(* Logix 5000 AddOnInstructionDefinition export FB_SCTMi_IOL; software revision 30.00 *)

TYPE stSCTMi_Ejector :
STRUCT
   siErrorByte : SINT;
   siWarningByte : SINT;
   siLeakageOfLastCycle : SINT;
   iSystemVacuum : INT;
   iEvacuationTimeT1 : INT;
   iLastFreeFlowVacuum : INT;
   iAirConsumptionOfLastCyc : INT;
   bAirSavingFunktion_H1 : BOOL;
   bPartPresent_H2 : BOOL;
END_STRUCT
END_TYPE

ADD_ON_INSTRUCTION FB_SCTMi_IOL   (* revision 1.0, vendor J. Schmalz GmbH *)
VAR_INPUT
   iInputPressure : INT; {access None, visible}
   bVacOnEjector1 : BOOL; {access None, visible}
   bBlowOffEjector1 : BOOL; {access None, visible}
   bVacOnEjector2 : BOOL; {access None, visible}
   bBlowOffEjector2 : BOOL; {access None, visible}
   bVacOnEjector3 : BOOL; {access None, visible}
   bBlowOffEjector3 : BOOL; {access None, visible}
   bVacOnEjector4 : BOOL; {access None, visible}
   bBlowOffEjector4 : BOOL; {access None, visible}
   bVacOnEjector5 : BOOL; {access None, visible}
   bBlowOffEjector5 : BOOL; {access None, visible}
   bVacOnEjector6 : BOOL; {access None, visible}
   bBlowOffEjector6 : BOOL; {access None, visible}
   bVacOnEjector7 : BOOL; {access None, visible}
   bBlowOffEjector7 : BOOL; {access None, visible}
   bVacOnEjector8 : BOOL; {access None, visible}
   bBlowOffEjector8 : BOOL; {access None, visible}
   bVacOnEjector9 : BOOL; {access None, visible}
   bBlowOffEjector9 : BOOL; {access None, visible}
   bVacOnEjector10 : BOOL; {access None, visible}
   bBlowOffEjector10 : BOOL; {access None, visible}
   bVacOnEjector11 : BOOL; {access None, visible}
   bBlowOffEjector11 : BOOL; {access None, visible}
   bVacOnEjector12 : BOOL; {access None, visible}
   bBlowOffEjector12 : BOOL; {access None, visible}
   bVacOnEjector13 : BOOL; {access None, visible}
   bBlowOffEjector13 : BOOL; {access None, visible}
   bVacOnEjector14 : BOOL; {access None, visible}
   bBlowOffEjector14 : BOOL; {access None, visible}
   bVacOnEjector15 : BOOL; {access None, visible}
   bBlowOffEjector15 : BOOL; {access None, visible}
   bVacOnEjector16 : BOOL; {access None, visible}
   bBlowOffEjector16 : BOOL; {access None, visible}
   iNumberOfEjectors : INT; {visible}
   iValveTypes : INT; {visible}
   siPDIData0 : SINT; {visible}
   siPDIData1 : SINT; {visible}
   siPDIData2 : SINT; {visible}
   siPDIData3 : SINT; {visible}
   siPDIData4 : SINT; {visible}
   siPDIData5 : SINT; {visible}
   siPDIData6 : SINT; {visible}
   siPDIData7 : SINT; {visible}
END_VAR
VAR_OUTPUT
   bDeviceStateGreen : BOOL; {visible}
   bDeviceStateYellow : BOOL; {visible}
   bDeviceStateOrange : BOOL; {visible}
   bDeviceStateRed : BOOL; {visible}
   siErrorByteCU : SINT; {visible}
   siWarningByteCU : SINT; {visible}
   iPrimSupplyVoltageCU : INT; {visible}
   iAuxSupplyVoltageCU : INT; {visible}
   iTotalAirConsCU : INT; {visible}
   siPDOData0 : SINT; {visible}
   siPDOData1 : SINT; {visible}
   siPDOData2 : SINT; {visible}
   siPDOData3 : SINT; {visible}
   siPDOData4 : SINT; {visible}
   siPDOData5 : SINT; {visible}
END_VAR
VAR_IN_OUT
   stDataEjector1To16 : stSCTMi_Ejector[16]; {required}
END_VAR
VAR
   iStep : INT; {access None}
   iBuffer0 : INT; {access None}
   iBuffer1 : INT; {access None}
END_VAR

ROUTINE Logic   (* structured text *)
   (*////////////////////////////////////////////////////////////////////////////////////////////////////////////////////////////////////////////////////////////////////
   // -------------------------------------------------------------------------------------------------------------------------------------------------------------------
   // Copyright (C) - J. Schmalz GmbH 2018 -  All rights reserved
   // Subject to change without notice
   // -------------------------------------------------------------------------------------------------------------------------------------------------------------------
   // This function block controls a Schmalz SCTMi-IOL via the process data. With this function block all possible
   // Combinations of ejectors can be controlled.
   // For further information on how the module must be parameterized can be found in the function block documentation.
   // -------------------------------------------------------------------------------------------------------------------------------------------------------------------
   // Version:			1.0
   // Issue Date:		2018-07-20
   // -------------------------------------------------------------------------------------------------------------------------------------------------------------------
   /////////////////////////////////////////////////////////////////////////////////////////////////////////////////////////////////////////////////////////////////////*)
   
   IF EnableIn THEN
   
   (*Sequence: Read epc values*)
   	CASE iStep OF
   
   (* Control Unit *)
   	0:
   		siPDOData0.0:=0;
   		siPDOData0.1:=0;
   		siPDOData0.2:=0;
   		siPDOData0.3:=0;
   		siPDOData0.4:=0;
   
   (* EPC-Value 0 *)
   		siPDOData0.6 := 0;
   		siPDOData0.7 := 0;
   		IF NOT siPDIData0.5  THEN
   			siErrorByteCU := siPDIData1;
   			iBuffer0 := siPDIData3;
   			iBuffer1 := siPDIData2 * 256;
   			iPrimSupplyVoltageCU := iBuffer1 OR iBuffer0;
   			iBuffer0 := 0;
   			iBuffer1 := 0;
   			iStep := iStep + 1;
   		END_IF;
   
   (* EPC-Value 1 *)
   	1:
   		siPDOData0.6 := 1;
   		siPDOData0.7 := 0;
   		IF siPDIData0.5  THEN
   			siWarningByteCU := siPDIData1;
   			iBuffer0 := siPDIData3;
   			iBuffer1 := siPDIData2 * 256;
   			iAuxSupplyVoltageCU := iBuffer1 OR iBuffer0;
   			iBuffer0 := 0;
   			iBuffer1 := 0;
   			iStep := iStep + 1;
   		END_IF;
   
   (* intermediate step *)
   	2:
   		siPDOData0.6 := 0;
   		siPDOData0.7 := 0;
   		IF NOT siPDIData0.5  THEN
   			iStep := iStep + 1;
   		END_IF;
   
   (* EPC-Value 2 *)
   	3:
   		siPDOData0.6 := 0;
   		siPDOData0.7 := 1;
   		IF siPDIData0.5  THEN
   			iStep := iStep + 1;
   		END_IF;
   
   (* intermediate step *)
   	4:
   		siPDOData0.6 := 0;
   		siPDOData0.7 := 0;
   		IF NOT siPDIData0.5  THEN
   			iStep := iStep + 1;
   		END_IF;
   
   (* EPC-Value 3 *)
   	5:
   		siPDOData0.6 := 1;
   		siPDOData0.7 := 1;
   		IF siPDIData0.5  THEN
   			iBuffer0 := siPDIData3;
   			iBuffer1 := siPDIData2 * 256;
   			iTotalAirConsCU := iBuffer1 OR iBuffer0;
   			iBuffer0 := 0;
   			iBuffer1 := 0;
   			iStep := iStep + 1;
   		END_IF;
   
   	6:
   			IF iNumberOfEjectors >= 1 THEN
   				iStep := iStep + 1;
   			ELSE
   				iStep:= 0;
   			END_IF;
   
   (* Ejector 1 *)
   	7:
   		siPDOData0.0:=1;
   		siPDOData0.1:=0;
   		siPDOData0.2:=0;
   		siPDOData0.3:=0;
   		siPDOData0.4:=0;
   
   (* EPC-Value 0 *)
   		siPDOData0.6 := 0;
   		siPDOData0.7 := 0;
   		IF NOT siPDIData0.5  THEN
   			stDataEjector1To16[0].siErrorByte := siPDIData1;
   			iBuffer0 := siPDIData3;
   			iBuffer1 := siPDIData2 * 256;
   			stDataEjector1To16[0].iSystemVacuum:= iBuffer1 OR iBuffer0;
   			iBuffer0 := 0;
   			iBuffer1 := 0;
   			iStep := iStep + 1;
   		END_IF;
   
   (* EPC-Value 1 *)
   	8:
   		siPDOData0.6 := 1;
   		siPDOData0.7 := 0;
   		IF siPDIData0.5  THEN
   			stDataEjector1To16[0].siWarningByte := siPDIData1;
   			iBuffer0 := siPDIData3;
   			iBuffer1 := siPDIData2 * 256;
   			stDataEjector1To16[0].iEvacuationTimeT1 := iBuffer1 OR iBuffer0;
   			iBuffer0 := 0;
   			iBuffer1 := 0;
   			iStep := iStep + 1;
   		END_IF;
   
   (* intermediate step *)
   	9:
   		siPDOData0.6 := 0;
   		siPDOData0.7 := 0;
   		IF NOT siPDIData0.5  THEN
   			iStep := iStep + 1;
   		END_IF;
   
   (* EPC-Value 2 *)
   	10:
   		siPDOData0.6 := 0;
   		siPDOData0.7 := 1;
   		IF siPDIData0.5  THEN
   			iBuffer0 := siPDIData3;
   			iBuffer1 := siPDIData2 * 256;
   			stDataEjector1To16[0].iLastFreeFlowVacuum := iBuffer1 OR iBuffer0;
   			iBuffer0 := 0;
   			iBuffer1 := 0;
   			iStep := iStep + 1;
   		END_IF;
   
   (* intermediate step *)
   	11:
   		siPDOData0.6 := 0;
   		siPDOData0.7 := 0;
   		IF NOT siPDIData0.5  THEN
   			iStep := iStep + 1;
   		END_IF;
   
    (* EPC-Value 3 *)
   	12:
   		siPDOData0.6 := 1;
   		siPDOData0.7 := 1;
   		IF siPDIData0.5  THEN
   			stDataEjector1To16[0].siLeakageOfLastCycle := siPDIData1;
   			iBuffer0 := siPDIData3;
   			iBuffer1 := siPDIData2 * 256;
   			stDataEjector1To16[0].iAirConsumptionOfLastCyc := iBuffer1 OR iBuffer0;
   			iBuffer0 := 0;
   			iBuffer1 := 0;
   			iStep := iStep + 1;
   		END_IF;
   
   	13:
   		IF iNumberOfEjectors >= 2 THEN
   			iStep := iStep + 1;
   		ELSE
   			iStep:= 0;
   		END_IF;
   
   (* Ejector 2 *)
   	14:
   		siPDOData0.0:=0;
   		siPDOData0.1:=1;
   		siPDOData0.2:=0;
   		siPDOData0.3:=0;
   		siPDOData0.4:=0;
   
   (* EPC-Value 0 *)
   		siPDOData0.6 := 0;
   		siPDOData0.7 := 0;
   		IF NOT siPDIData0.5  THEN
   			stDataEjector1To16[1].siErrorByte := siPDIData1;
   			iBuffer0 := siPDIData3;
   			iBuffer1 := siPDIData2 * 256;
   			stDataEjector1To16[1].iSystemVacuum:= iBuffer1 OR iBuffer0;
   			iBuffer0 := 0;
   			iBuffer1 := 0;
   			iStep := iStep + 1;
   		END_IF;
   
   (* EPC-Value 1 *)
   	15:
   		siPDOData0.6 := 1;
   		siPDOData0.7 := 0;
   		IF siPDIData0.5  THEN
   			stDataEjector1To16[1].siWarningByte := siPDIData1;
   			iBuffer0 := siPDIData3;
   			iBuffer1 := siPDIData2 * 256;
   			stDataEjector1To16[1].iEvacuationTimeT1 := iBuffer1 OR iBuffer0;
   			iBuffer0 := 0;
   			iBuffer1 := 0;
   			iStep := iStep + 1;
   		END_IF;
   
   (* intermediate step *)
   	16:
   		siPDOData0.6 := 0;
   		siPDOData0.7 := 0;
   		IF NOT siPDIData0.5  THEN
   			iStep := iStep + 1;
   		END_IF;
   
   (* EPC-Value 2 *)
   	17:
   		siPDOData0.6 := 0;
   		siPDOData0.7 := 1;
   		IF siPDIData0.5  THEN
   			iBuffer0 := siPDIData3;
   			iBuffer1 := siPDIData2 * 256;
   			stDataEjector1To16[1].iLastFreeFlowVacuum := iBuffer1 OR iBuffer0;
   			iBuffer0 := 0;
   			iBuffer1 := 0;
   			iStep := iStep + 1;
   		END_IF;
   
   (* intermediate step *)
   	18:
   		siPDOData0.6 := 0;
   		siPDOData0.7 := 0;
   		IF NOT siPDIData0.5  THEN
   			iStep := iStep + 1;
   		END_IF;
   
   (* EPC-Value 3 *)
   	19:	(* EPC-Value 3 *)
   		siPDOData0.6 := 1;
   		siPDOData0.7 := 1;
   		IF siPDIData0.5  THEN
   			stDataEjector1To16[1].siLeakageOfLastCycle := siPDIData1;
   			iBuffer0 := siPDIData3;
   			iBuffer1 := siPDIData2 * 256;
   			stDataEjector1To16[1].iAirConsumptionOfLastCyc := iBuffer1 OR iBuffer0;
   			iBuffer0 := 0;
   			iBuffer1 := 0;
   			iStep := iStep + 1;
   		END_IF;
   
   	20:
   		IF iNumberOfEjectors >= 3 THEN
   			iStep := iStep + 1;
   		ELSE
   			iStep:= 0;
   		END_IF;
   
   (* Ejector 3 *)
   	21:
   		siPDOData0.0:=1;
   		siPDOData0.1:=1;
   		siPDOData0.2:=0;
   		siPDOData0.3:=0;
   		siPDOData0.4:=0;
   
   (* EPC-Value 0 *)
   		siPDOData0.6 := 0;
   		siPDOData0.7 := 0;
   		IF NOT siPDIData0.5  THEN
   			stDataEjector1To16[2].siErrorByte := siPDIData1;
   			iBuffer0 := siPDIData3;
   			iBuffer1 := siPDIData2 * 256;
   			stDataEjector1To16[2].iSystemVacuum:= iBuffer1 OR iBuffer0;
   			iBuffer0 := 0;
   			iBuffer1 := 0;
   			iStep := iStep + 1;
   		END_IF;
   
   (* EPC-Value 1 *)
   	22:
   		siPDOData0.6 := 1;
   		siPDOData0.7 := 0;
   		IF siPDIData0.5  THEN
   			stDataEjector1To16[2].siWarningByte := siPDIData1;
   			iBuffer0 := siPDIData3;
   			iBuffer1 := siPDIData2 * 256;
   			stDataEjector1To16[2].iEvacuationTimeT1 := iBuffer1 OR iBuffer0;
   			iBuffer0 := 0;
   			iBuffer1 := 0;
   			iStep := iStep + 1;
   		END_IF;
   
   (* intermediate step *)
   	23:
   		siPDOData0.6 := 0;
   		siPDOData0.7 := 0;
   		IF NOT siPDIData0.5  THEN
   			iStep := iStep + 1;
   		END_IF;
   
   (* EPC-Value 2 *)
   	24:
   		siPDOData0.6 := 0;
   		siPDOData0.7 := 1;
   		IF siPDIData0.5  THEN
   			iBuffer0 := siPDIData3;
   			iBuffer1 := siPDIData2 * 256;
   			stDataEjector1To16[2].iLastFreeFlowVacuum := iBuffer1 OR iBuffer0;
   			iBuffer0 := 0;
   			iBuffer1 := 0;
   			iStep := iStep + 1;
   		END_IF;
   
   (* intermediate step *)
   	25:
   		siPDOData0.6 := 0;
   		siPDOData0.7 := 0;
   		IF NOT siPDIData0.5  THEN
   			iStep := iStep + 1;
   		END_IF;
   
   (* EPC-Value 3 *)
   	26:
   		siPDOData0.6 := 1;
   		siPDOData0.7 := 1;
   		IF siPDIData0.5  THEN
   			stDataEjector1To16[2].siLeakageOfLastCycle := siPDIData1;
   			iBuffer0 := siPDIData3;
   			iBuffer1 := siPDIData2 * 256;
   			stDataEjector1To16[2].iAirConsumptionOfLastCyc := iBuffer1 OR iBuffer0;
   			iBuffer0 := 0;
   			iBuffer1 := 0;
   			iStep := iStep + 1;
   		END_IF;
   
   	27:
   		IF iNumberOfEjectors >= 4 THEN
   			iStep := iStep + 1;
   		ELSE
   			iStep:= 0;
   		END_IF;
   
   (* Ejector 4 *)
   	28:
   		siPDOData0.0:=0;
   		siPDOData0.1:=0;
   		siPDOData0.2:=1;
   		siPDOData0.3:=0;
   		siPDOData0.4:=0;
   
   (* EPC-Value 0 *)
   		siPDOData0.6 := 0;
   		siPDOData0.7 := 0;
   		IF NOT siPDIData0.5  THEN
   			stDataEjector1To16[3].siErrorByte := siPDIData1;
   			iBuffer0 := siPDIData3;
   			iBuffer1 := siPDIData2 * 256;
   			stDataEjector1To16[3].iSystemVacuum := iBuffer1 OR iBuffer0;
   			iBuffer0 := 0;
   			iBuffer1 := 0;
   			iStep := iStep + 1;
   		END_IF;
   
   (* EPC-Value 1 *)
   	29:
   		siPDOData0.6 := 1;
   		siPDOData0.7 := 0;
   		IF siPDIData0.5  THEN
   			stDataEjector1To16[3].siWarningByte := siPDIData1;
   			iBuffer0 := siPDIData3;
   			iBuffer1 := siPDIData2 * 256;
   			stDataEjector1To16[3].iEvacuationTimeT1 := iBuffer1 OR iBuffer0;
   			iBuffer0 := 0;
   			iBuffer1 := 0;
   			iStep := iStep + 1;
   		END_IF;
   
   (* intermediate step *)
   	30:
   		siPDOData0.6 := 0;
   		siPDOData0.7 := 0;
   		IF NOT siPDIData0.5  THEN
   			iStep := iStep + 1;
   		END_IF;
   
   (* EPC-Value 2 *)
   	31:
   		siPDOData0.6 := 0;
   		siPDOData0.7 := 1;
   		IF siPDIData0.5  THEN
   			iBuffer0 := siPDIData3;
   			iBuffer1 := siPDIData2 * 256;
   			stDataEjector1To16[3].iLastFreeFlowVacuum := iBuffer1 OR iBuffer0;
   			iBuffer0 := 0;
   			iBuffer1 := 0;
   			iStep := iStep + 1;
   		END_IF;
   
   (* intermediate step *)
   	32:
   		siPDOData0.6 := 0;
   		siPDOData0.7 := 0;
   		IF NOT siPDIData0.5  THEN
   			iStep := iStep + 1;
   		END_IF;
   
   (* EPC-Value 3 *)
   	33:
   		siPDOData0.6 := 1;
   		siPDOData0.7 := 1;
   		IF siPDIData0.5  THEN
   			stDataEjector1To16[3].siLeakageOfLastCycle := siPDIData1;
   			iBuffer0 := siPDIData3;
   			iBuffer1 := siPDIData2 * 256;
   			stDataEjector1To16[3].iAirConsumptionOfLastCyc := iBuffer1 OR iBuffer0;
   			iBuffer0 := 0;
   			iBuffer1 := 0;
   			iStep := iStep + 1;
   		END_IF;
   
   	34:
   		IF iNumberOfEjectors >= 5 THEN
   			iStep := iStep + 1;
   		ELSE
   			iStep:= 0;
   		END_IF;
   
   
   (* Ejector 5 *)
   	35:
   		siPDOData0.0:=1;
   		siPDOData0.1:=0;
   		siPDOData0.2:=1;
   		siPDOData0.3:=0;
   		siPDOData0.4:=0;
   
   (* EPC-Value 0 *)
   		siPDOData0.6 := 0;
   		siPDOData0.7 := 0;
   		IF NOT siPDIData0.5  THEN
   			stDataEjector1To16[4].siErrorByte := siPDIData1;
   			iBuffer0 := siPDIData3;
   			iBuffer1 := siPDIData2 * 256;
   			stDataEjector1To16[4].iSystemVacuum:= iBuffer1 OR iBuffer0;
   			iBuffer0 := 0;
   			iBuffer1 := 0;
   			iStep := iStep + 1;
   		END_IF;
   
   (* EPC-Value 1 *)
   	36:
   		siPDOData0.6 := 1;
   		siPDOData0.7 := 0;
   		IF siPDIData0.5  THEN
   			stDataEjector1To16[4].siWarningByte := siPDIData1;
   			iBuffer0 := siPDIData3;
   			iBuffer1 := siPDIData2 * 256;
   			stDataEjector1To16[4].iEvacuationTimeT1 := iBuffer1 OR iBuffer0;
   			iBuffer0 := 0;
   			iBuffer1 := 0;
   			iStep := iStep + 1;
   		END_IF;
   
   (* intermediate step *)
   	37:
   		siPDOData0.6 := 0;
   		siPDOData0.7 := 0;
   		IF NOT siPDIData0.5  THEN
   			iStep := iStep + 1;
   		END_IF;
   
   (* EPC-Value 2 *)
   	38:
   		siPDOData0.6 := 0;
   		siPDOData0.7 := 1;
   		IF siPDIData0.5  THEN
   			iBuffer0 := siPDIData3;
   			iBuffer1 := siPDIData2 * 256;
   			stDataEjector1To16[4].iLastFreeFlowVacuum := iBuffer1 OR iBuffer0;
   			iBuffer0 := 0;
   			iBuffer1 := 0;
   			iStep := iStep + 1;
   		END_IF;
   
   (* intermediate step *)
   	39:
   		siPDOData0.6 := 0;
   		siPDOData0.7 := 0;
   		IF NOT siPDIData0.5  THEN
   			iStep := iStep + 1;
   		END_IF;
   
   (* EPC-Value 3 *)
   	40:
   		siPDOData0.6 := 1;
   		siPDOData0.7 := 1;
   		IF siPDIData0.5  THEN
   			stDataEjector1To16[4].siLeakageOfLastCycle := siPDIData1;
   			iBuffer0 := siPDIData3;
   			iBuffer1 := siPDIData2 * 256;
   			stDataEjector1To16[4].iAirConsumptionOfLastCyc := iBuffer1 OR iBuffer0;
   			iBuffer0 := 0;
   			iBuffer1 := 0;
   			iStep := iStep + 1;
   		END_IF;
   
   	41:
   		IF iNumberOfEjectors >= 6 THEN
   			iStep := iStep + 1;
   		ELSE
   			iStep:= 0;
   		END_IF;
   
   (* Ejector 6 *)
   	42:
   		siPDOData0.0:=0;
   		siPDOData0.1:=1;
   		siPDOData0.2:=1;
   		siPDOData0.3:=0;
   		siPDOData0.4:=0;
   
   (* EPC-Value 0 *)
   		siPDOData0.6 := 0;
   		siPDOData0.7 := 0;
   		IF NOT siPDIData0.5  THEN
   			stDataEjector1To16[5].siErrorByte := siPDIData1;
   			iBuffer0 := siPDIData3;
   			iBuffer1 := siPDIData2 * 256;
   			stDataEjector1To16[5].iSystemVacuum:= iBuffer1 OR iBuffer0;
   			iBuffer0 := 0;
   			iBuffer1 := 0;
   			iStep := iStep + 1;
   		END_IF;
   
   (* EPC-Value 1 *)
   	43:
   		siPDOData0.6 := 1;
   		siPDOData0.7 := 0;
   		IF siPDIData0.5  THEN
   			stDataEjector1To16[5].siWarningByte := siPDIData1;
   			iBuffer0 := siPDIData3;
   			iBuffer1 := siPDIData2 * 256;
   			stDataEjector1To16[5].iEvacuationTimeT1 := iBuffer1 OR iBuffer0;
   			iBuffer0 := 0;
   			iBuffer1 := 0;
   			iStep := iStep + 1;
   		END_IF;
   
   (* intermediate step *)
   	44:
   		siPDOData0.6 := 0;
   		siPDOData0.7 := 0;
   
   		IF NOT siPDIData0.5  THEN
   			iStep := iStep + 1;
   		END_IF;
   
   (* EPC-Value 2 *)
   	45:
   		siPDOData0.6 := 0;
   		siPDOData0.7 := 1;
   		IF siPDIData0.5  THEN
   			iBuffer0 := siPDIData3;
   			iBuffer1 := siPDIData2 * 256;
   			stDataEjector1To16[5].iLastFreeFlowVacuum := iBuffer1 OR iBuffer0;
   			iBuffer0 := 0;
   			iBuffer1 := 0;
   			iStep := iStep + 1;
   		END_IF;
   
   (* intermediate step *)
   	46:
   		siPDOData0.6 := 0;
   		siPDOData0.7 := 0;
   		IF NOT siPDIData0.5  THEN
   			iStep := iStep + 1;
   		END_IF;
   
   (* EPC-Value 3 *)
   	47:
   		siPDOData0.6 := 1;
   		siPDOData0.7 := 1;
   		IF siPDIData0.5  THEN
   			stDataEjector1To16[5].siLeakageOfLastCycle := siPDIData1;
   			iBuffer0 := siPDIData3;
   			iBuffer1 := siPDIData2 * 256;
   			stDataEjector1To16[5].iAirConsumptionOfLastCyc := iBuffer1 OR iBuffer0;
   			iBuffer0 := 0;
   			iBuffer1 := 0;
   			iStep := iStep + 1;
   		END_IF;
   
   	48:
   		IF iNumberOfEjectors >= 7 THEN
   			iStep := iStep + 1;
   		ELSE
   			iStep:= 0;
   		END_IF;
   
   (* Ejector 7 *)
   	49:
   		siPDOData0.0:=1;
   		siPDOData0.1:=1;
   		siPDOData0.2:=1;
   		siPDOData0.3:=0;
   		siPDOData0.4:=0;
   
   (* EPC-Value 0 *)
   		siPDOData0.6 := 0;
   		siPDOData0.7 := 0;
   		IF NOT siPDIData0.5  THEN
   			stDataEjector1To16[6].siErrorByte := siPDIData1;
   			iBuffer0 := siPDIData3;
   			iBuffer1 := siPDIData2 * 256;
   			stDataEjector1To16[6].iSystemVacuum:= iBuffer1 OR iBuffer0;
   			iBuffer0 := 0;
   			iBuffer1 := 0;
   			iStep := iStep + 1;
   		END_IF;
   
   (* EPC-Value 1 *)
   	50:
   		siPDOData0.6 := 1;
   		siPDOData0.7 := 0;
   		IF siPDIData0.5  THEN
   			stDataEjector1To16[6].siWarningByte := siPDIData1;
   			iBuffer0 := siPDIData3;
   			iBuffer1 := siPDIData2 * 256;
   			stDataEjector1To16[6].iEvacuationTimeT1 := iBuffer1 OR iBuffer0;
   			iBuffer0 := 0;
   			iBuffer1 := 0;
   			iStep := iStep + 1;
   		END_IF;
   
   (* intermediate step *)
   	51:
   		siPDOData0.6 := 0;
   		siPDOData0.7 := 0;
   		IF NOT siPDIData0.5  THEN
   			iStep := iStep + 1;
   		END_IF;
   
   (* EPC-Value 2 *)
   	52:
   		siPDOData0.6 := 0;
   		siPDOData0.7 := 1;
   		IF siPDIData0.5  THEN
   			iBuffer0 := siPDIData3;
   			iBuffer1 := siPDIData2 * 256;
   			stDataEjector1To16[6].iLastFreeFlowVacuum := iBuffer1 OR iBuffer0;
   			iBuffer0 := 0;
   			iBuffer1 := 0;
   			iStep := iStep + 1;
   		END_IF;
   
   (* intermediate step *)
   	53:
   		siPDOData0.6 := 0;
   		siPDOData0.7 := 0;
   		IF NOT siPDIData0.5  THEN
   			iStep := iStep + 1;
   		END_IF;
   
   (* EPC-Value 3 *)
   	54:
   		siPDOData0.6 := 1;
   		siPDOData0.7 := 1;
   		IF siPDIData0.5  THEN
   			stDataEjector1To16[6].siLeakageOfLastCycle := siPDIData1;
   			iBuffer0 := siPDIData3;
   			iBuffer1 := siPDIData2 * 256;
   			stDataEjector1To16[6].iAirConsumptionOfLastCyc := iBuffer1 OR iBuffer0;
   			iBuffer0 := 0;
   			iBuffer1 := 0;
   			iStep := iStep + 1;
   		END_IF;
   
   	55:
   		IF iNumberOfEjectors >= 8 THEN
   			iStep := iStep + 1;
   		ELSE
   			iStep:= 0;
   		END_IF;
   
   (* Ejector 8 *)
   	56:
   		siPDOData0.0:=0;
   		siPDOData0.1:=0;
   		siPDOData0.2:=0;
   		siPDOData0.3:=1;
   		siPDOData0.4:=0;
   
   (* EPC-Value 0 *)
   		siPDOData0.6 := 0;
   		siPDOData0.7 := 0;
   		IF NOT siPDIData0.5  THEN
   			stDataEjector1To16[7].siErrorByte := siPDIData1;
   			iBuffer0 := siPDIData3;
   			iBuffer1 := siPDIData2 * 256;
   			stDataEjector1To16[7].iSystemVacuum:= iBuffer1 OR iBuffer0;
   			iBuffer0 := 0;
   			iBuffer1 := 0;
   			iStep := iStep + 1;
   		END_IF;
   
   (* EPC-Value 1 *)
   	57:
   		siPDOData0.6 := 1;
   		siPDOData0.7 := 0;
   		IF siPDIData0.5  THEN
   			stDataEjector1To16[7].siWarningByte := siPDIData1;
   			iBuffer0 := siPDIData3;
   			iBuffer1 := siPDIData2 * 256;
   			stDataEjector1To16[7].iEvacuationTimeT1 := iBuffer1 OR iBuffer0;
   			iBuffer0 := 0;
   			iBuffer1 := 0;
   			iStep := iStep + 1;
   		END_IF;
   
   (* intermediate step *)
   	58:
   		siPDOData0.6 := 0;
   		siPDOData0.7 := 0;
   		IF NOT siPDIData0.5  THEN
   			iStep := iStep + 1;
   		END_IF;
   
   (* EPC-Value 2 *)
   	59:
   		siPDOData0.6 := 0;
   		siPDOData0.7 := 1;
   		IF siPDIData0.5  THEN
   			iBuffer0 := siPDIData3;
   			iBuffer1 := siPDIData2 * 256;
   			stDataEjector1To16[7].iLastFreeFlowVacuum := iBuffer1 OR iBuffer0;
   			iBuffer0 := 0;
   			iBuffer1 := 0;
   			iStep := iStep + 1;
   		END_IF;
   
   (* intermediate step *)
   	60:
   		siPDOData0.6 := 0;
   		siPDOData0.7 := 0;
   		IF NOT siPDIData0.5  THEN
   			iStep := iStep + 1;
   		END_IF;
   
   (* EPC-Value 3 *)
   	61:
   		siPDOData0.6 := 1;
   		siPDOData0.7 := 1;
   		IF siPDIData0.5  THEN
   			stDataEjector1To16[7].siLeakageOfLastCycle := siPDIData1;
   			iBuffer0 := siPDIData3;
   			iBuffer1 := siPDIData2 * 256;
   			stDataEjector1To16[7].iAirConsumptionOfLastCyc := iBuffer1 OR iBuffer0;
   			iBuffer0 := 0;
   			iBuffer1 := 0;
   			iStep := iStep + 1;
   		END_IF;
   
   	62:
   		IF iNumberOfEjectors >= 9 THEN
   			iStep := iStep + 1;
   		ELSE
   			iStep:= 0;
   		END_IF;
   
   (* Ejector 9 *)
   	63:
   		siPDOData0.0:=1;
   		siPDOData0.1:=0;
   		siPDOData0.2:=0;
   		siPDOData0.3:=1;
   		siPDOData0.4:=0;
   
   (* EPC-Value 0 *)
   		siPDOData0.6 := 0;
   		siPDOData0.7 := 0;
   		IF NOT siPDIData0.5  THEN
   			stDataEjector1To16[8].siErrorByte := siPDIData1;
   			iBuffer0 := siPDIData3;
   			iBuffer1 := siPDIData2 * 256;
   			stDataEjector1To16[8].iSystemVacuum:= iBuffer1 OR iBuffer0;
   			iBuffer0 := 0;
   			iBuffer1 := 0;
   			iStep := iStep + 1;
   		END_IF;
   
   (* EPC-Value 1 *)
   	64:
   		siPDOData0.6 := 1;
   		siPDOData0.7 := 0;
   		IF siPDIData0.5  THEN
   			stDataEjector1To16[8].siWarningByte := siPDIData1;
   			iBuffer0 := siPDIData3;
   			iBuffer1 := siPDIData2 * 256;
   			stDataEjector1To16[8].iEvacuationTimeT1 := iBuffer1 OR iBuffer0;
   			iBuffer0 := 0;
   			iBuffer1 := 0;
   			iStep := iStep + 1;
   		END_IF;
   
   (* intermediate step *)
   	65:
   		siPDOData0.6 := 0;
   		siPDOData0.7 := 0;
   		IF NOT siPDIData0.5  THEN
   			iStep := iStep + 1;
   		END_IF;
   
   (* EPC-Value 2 *)
   	66:
   		siPDOData0.6 := 0;
   		siPDOData0.7 := 1;
   		IF siPDIData0.5  THEN
   			iBuffer0 := siPDIData3;
   			iBuffer1 := siPDIData2 * 256;
   			stDataEjector1To16[8].iLastFreeFlowVacuum := iBuffer1 OR iBuffer0;
   			iBuffer0 := 0;
   			iBuffer1 := 0;
   			iStep := iStep + 1;
   		END_IF;
   
   (* intermediate step *)
   	67:
   		siPDOData0.6 := 0;
   		siPDOData0.7 := 0;
   		IF NOT siPDIData0.5  THEN
   			iStep := iStep + 1;
   		END_IF;
   
   (* EPC-Value 3 *)
   	68:
   		siPDOData0.6 := 1;
   		siPDOData0.7 := 1;
   		IF siPDIData0.5  THEN
   			stDataEjector1To16[8].siLeakageOfLastCycle := siPDIData1;
   			iBuffer0 := siPDIData3;
   			iBuffer1 := siPDIData2 * 256;
   			stDataEjector1To16[8].iAirConsumptionOfLastCyc := iBuffer1 OR iBuffer0;
   			iBuffer0 := 0;
   			iBuffer1 := 0;
   			iStep := iStep + 1;
   		END_IF;
   
   	69:
   		IF iNumberOfEjectors >= 10 THEN
   			iStep := iStep + 1;
   		ELSE
   			iStep:= 0;
   		END_IF;
   
   (* Ejector 10 *)
   
   	70:
   		siPDOData0.0:=0;
   		siPDOData0.1:=1;
   		siPDOData0.2:=0;
   		siPDOData0.3:=1;
   		siPDOData0.4:=0;
   
   (* EPC-Value 0 *)
   		siPDOData0.6 := 0;
   		siPDOData0.7 := 0;
   		IF NOT siPDIData0.5  THEN
   			stDataEjector1To16[9].siErrorByte := siPDIData1;
   			iBuffer0 := siPDIData3;
   			iBuffer1 := siPDIData2 * 256;
   			stDataEjector1To16[9].iSystemVacuum:= iBuffer1 OR iBuffer0;
   			iBuffer0 := 0;
   			iBuffer1 := 0;
   			iStep := iStep + 1;
   		END_IF;
   
   (* EPC-Value 1 *)
   	71:
   		siPDOData0.6 := 1;
   		siPDOData0.7 := 0;
   		IF siPDIData0.5  THEN
   			stDataEjector1To16[9].siWarningByte := siPDIData1;
   			iBuffer0 := siPDIData3;
   			iBuffer1 := siPDIData2 * 256;
   			stDataEjector1To16[9].iEvacuationTimeT1 := iBuffer1 OR iBuffer0;
   			iBuffer0 := 0;
   			iBuffer1 := 0;
   			iStep := iStep + 1;
   		END_IF;
   
   (* intermediate step *)
   	72:
   		siPDOData0.6 := 0;
   		siPDOData0.7 := 0;
   		IF NOT siPDIData0.5  THEN
   			iStep := iStep + 1;
   		END_IF;
   
   (* EPC-Value 2 *)
   	73:
   		siPDOData0.6 := 0;
   		siPDOData0.7 := 1;
   		IF siPDIData0.5  THEN
   			iBuffer0 := siPDIData3;
   			iBuffer1 := siPDIData2 * 256;
   			stDataEjector1To16[9].iLastFreeFlowVacuum := iBuffer1 OR iBuffer0;
   			iBuffer0 := 0;
   			iBuffer1 := 0;
   			iStep := iStep + 1;
   		END_IF;
   
   (* intermediate step *)
   	74:
   		siPDOData0.6 := 0;
   		siPDOData0.7 := 0;
   		IF NOT siPDIData0.5  THEN
   			iStep := iStep + 1;
   		END_IF;
   
   (* EPC-Value 3 *)
   	75:
   		siPDOData0.6 := 1;
   		siPDOData0.7 := 1;
   		IF siPDIData0.5  THEN
   			stDataEjector1To16[9].siLeakageOfLastCycle := siPDIData1;
   			iBuffer0 := siPDIData3;
   			iBuffer1 := siPDIData2 * 256;
   			stDataEjector1To16[9].iAirConsumptionOfLastCyc := iBuffer1 OR iBuffer0;
   			iBuffer0 := 0;
   			iBuffer1 := 0;
   			iStep := iStep + 1;
   		END_IF;
   
   	76:
   		IF iNumberOfEjectors >= 11 THEN
   			iStep := iStep + 1;
   		ELSE
   			iStep:= 0;
   		END_IF;
   
   (* Ejector 11 *)
   	77:
   		siPDOData0.0:=1;
   		siPDOData0.1:=1;
   		siPDOData0.2:=0;
   		siPDOData0.3:=1;
   		siPDOData0.4:=0;
   
   (* EPC-Value 0 *)
   		siPDOData0.6 := 0;
   		siPDOData0.7 := 0;
   		IF NOT siPDIData0.5  THEN
   			stDataEjector1To16[10].siErrorByte := siPDIData1;
   			iBuffer0 := siPDIData3;
   			iBuffer1 := siPDIData2 * 256;
   			stDataEjector1To16[10].iSystemVacuum:= iBuffer1 OR iBuffer0;
   			iBuffer0 := 0;
   			iBuffer1 := 0;
   			iStep := iStep + 1;
   		END_IF;
   
   (* EPC-Value 1 *)
   	78:
   		siPDOData0.6 := 1;
   		siPDOData0.7 := 0;
   		IF siPDIData0.5  THEN
   			stDataEjector1To16[10].siWarningByte := siPDIData1;
   			iBuffer0 := siPDIData3;
   			iBuffer1 := siPDIData2 * 256;
   			stDataEjector1To16[10].iEvacuationTimeT1 := iBuffer1 OR iBuffer0;
   			iBuffer0 := 0;
   			iBuffer1 := 0;
   			iStep := iStep + 1;
   		END_IF;
   
   (* intermediate step *)
   	79:
   		siPDOData0.6 := 0;
   		siPDOData0.7 := 0;
   		IF NOT siPDIData0.5  THEN
   			iStep := iStep + 1;
   		END_IF;
   
   (* EPC-Value 2 *)
   	80:
   		siPDOData0.6 := 0;
   		siPDOData0.7 := 1;
   		IF siPDIData0.5  THEN
   			iBuffer0 := siPDIData3;
   			iBuffer1 := siPDIData2 * 256;
   			stDataEjector1To16[10].iLastFreeFlowVacuum := iBuffer1 OR iBuffer0;
   			iBuffer0 := 0;
   			iBuffer1 := 0;
   			iStep := iStep + 1;
   		END_IF;
   
   (* intermediate step *)
   	81:
   		siPDOData0.6 := 0;
   		siPDOData0.7 := 0;
   		IF NOT siPDIData0.5  THEN
   			iStep := iStep + 1;
   		END_IF;
   
   (* EPC-Value 3 *)
   	82:
   		siPDOData0.6 := 1;
   		siPDOData0.7 := 1;
   		IF siPDIData0.5  THEN
   			stDataEjector1To16[10].siLeakageOfLastCycle := siPDIData1;
   			iBuffer0 := siPDIData3;
   			iBuffer1 := siPDIData2 * 256;
   			stDataEjector1To16[10].iAirConsumptionOfLastCyc := iBuffer1 OR iBuffer0;
   			iBuffer0 := 0;
   			iBuffer1 := 0;
   			iStep := iStep + 1;
   		END_IF;
   
   	83:
   		IF iNumberOfEjectors >= 12 THEN
   			iStep := iStep + 1;
   		ELSE
   			iStep:= 0;
   		END_IF;
   
   (* Ejector 12 *)
   	84:
   		siPDOData0.0:=0;
   		siPDOData0.1:=0;
   		siPDOData0.2:=1;
   		siPDOData0.3:=1;
   		siPDOData0.4:=0;
   
   (* EPC-Value 0 *)
   		siPDOData0.6 := 0;
   		siPDOData0.7 := 0;
   		IF NOT siPDIData0.5  THEN
   			stDataEjector1To16[11].siErrorByte := siPDIData1;
   			iBuffer0 := siPDIData3;
   			iBuffer1 := siPDIData2 * 256;
   			stDataEjector1To16[11].iSystemVacuum:= iBuffer1 OR iBuffer0;
   			iBuffer0 := 0;
   			iBuffer1 := 0;
   			iStep := iStep + 1;
   		END_IF;
   
   (* EPC-Value 1 *)
   	85:
   		siPDOData0.6 := 1;
   		siPDOData0.7 := 0;
   		IF siPDIData0.5  THEN
   			stDataEjector1To16[11].siWarningByte := siPDIData1;
   			iBuffer0 := siPDIData3;
   			iBuffer1 := siPDIData2 * 256;
   			stDataEjector1To16[11].iEvacuationTimeT1 := iBuffer1 OR iBuffer0;
   			iBuffer0 := 0;
   			iBuffer1 := 0;
   			iStep := iStep + 1;
   		END_IF;
   
   (* intermediate step *)
   	86:
   		siPDOData0.6 := 0;
   		siPDOData0.7 := 0;
   		IF NOT siPDIData0.5  THEN
   			iStep := iStep + 1;
   		END_IF;
   
   (* EPC-Value 2 *)
   	87:
   		siPDOData0.6 := 0;
   		siPDOData0.7 := 1;
   		IF siPDIData0.5  THEN
   			iBuffer0 := siPDIData3;
   			iBuffer1 := siPDIData2 * 256;
   			stDataEjector1To16[11].iLastFreeFlowVacuum := iBuffer1 OR iBuffer0;
   			iBuffer0 := 0;
   			iBuffer1 := 0;
   			iStep := iStep + 1;
   		END_IF;
   
   (* intermediate step *)
   	88:
   		siPDOData0.6 := 0;
   		siPDOData0.7 := 0;
   		IF NOT siPDIData0.5  THEN
   			iStep := iStep + 1;
   		END_IF;
   
   (* EPC-Value 3 *)
   	89:
   		siPDOData0.6 := 1;
   		siPDOData0.7 := 1;
   		IF siPDIData0.5  THEN
   			stDataEjector1To16[11].siLeakageOfLastCycle := siPDIData1;
   			iBuffer0 := siPDIData3;
   			iBuffer1 := siPDIData2 * 256;
   			stDataEjector1To16[11].iAirConsumptionOfLastCyc := iBuffer1 OR iBuffer0;
   			iBuffer0 := 0;
   			iBuffer1 := 0;
   			iStep := iStep + 1;
   		END_IF;
   
   	90:
   		IF iNumberOfEjectors >= 13 THEN
   			iStep := iStep + 1;
   		ELSE
   			iStep:= 0;
   		END_IF;
   
   (* Ejector 13 *)
   	91:
   		siPDOData0.0:=1;
   		siPDOData0.1:=0;
   		siPDOData0.2:=1;
   		siPDOData0.3:=1;
   		siPDOData0.4:=0;
   
   (* EPC-Value 0 *)
   		siPDOData0.6 := 0;
   		siPDOData0.7 := 0;
   		IF NOT siPDIData0.5  THEN
   			stDataEjector1To16[12].siErrorByte := siPDIData1;
   			iBuffer0 := siPDIData3;
   			iBuffer1 := siPDIData2 * 256;
   			stDataEjector1To16[12].iSystemVacuum:= iBuffer1 OR iBuffer0;
   			iBuffer0 := 0;
   			iBuffer1 := 0;
   			iStep := iStep + 1;
   		END_IF;
   
   (* EPC-Value 1 *)
   	92:
   		siPDOData0.6 := 1;
   		siPDOData0.7 := 0;
   		IF siPDIData0.5  THEN
   			stDataEjector1To16[12].siWarningByte := siPDIData1;
   			iBuffer0 := siPDIData3;
   			iBuffer1 := siPDIData2 * 256;
   			stDataEjector1To16[12].iEvacuationTimeT1 := iBuffer1 OR iBuffer0;
   			iBuffer0 := 0;
   			iBuffer1 := 0;
   			iStep := iStep + 1;
   		END_IF;
   
   (* intermediate step *)
   	93:
   		siPDOData0.6 := 0;
   		siPDOData0.7 := 0;
   		IF NOT siPDIData0.5  THEN
   			iStep := iStep + 1;
   		END_IF;
   
   (* EPC-Value 2 *)
   	94:
   		siPDOData0.6 := 0;
   		siPDOData0.7 := 1;
   		IF siPDIData0.5  THEN
   		iBuffer0 := siPDIData3;
   			iBuffer1 := siPDIData2 * 256;
   			stDataEjector1To16[12].iLastFreeFlowVacuum := iBuffer1 OR iBuffer0;
   			iBuffer0 := 0;
   			iBuffer1 := 0;
   			iStep := iStep + 1;
   		END_IF;
   
   (* intermediate step *)
   	95:
   		siPDOData0.6 := 0;
   		siPDOData0.7 := 0;
   		IF NOT siPDIData0.5  THEN
   			iStep := iStep + 1;
   		END_IF;
   
   (* EPC-Value 3 *)
   	96:
   		siPDOData0.6 := 1;
   		siPDOData0.7 := 1;
   		IF siPDIData0.5  THEN
   			stDataEjector1To16[12].siLeakageOfLastCycle := siPDIData1;
   			iBuffer0 := siPDIData3;
   			iBuffer1 := siPDIData2 * 256;
   			stDataEjector1To16[12].iAirConsumptionOfLastCyc := iBuffer1 OR iBuffer0;
   			iBuffer0 := 0;
   			iBuffer1 := 0;
   			iStep := iStep + 1;
   		END_IF;
   
   	97:
   		IF iNumberOfEjectors >= 14 THEN
   			iStep := iStep + 1;
   		ELSE
   			iStep:= 0;
   		END_IF;
   
   (* Ejector 14 *)
   	98:
   		siPDOData0.0:=0;
   		siPDOData0.1:=1;
   		siPDOData0.2:=1;
   		siPDOData0.3:=1;
   		siPDOData0.4:=0;
   
   (* EPC-Value 0 *)
   		siPDOData0.6 := 0;
   		siPDOData0.7 := 0;
   		IF NOT siPDIData0.5  THEN
   			stDataEjector1To16[13].siErrorByte := siPDIData1;
   			iBuffer0 := siPDIData3;
   			iBuffer1 := siPDIData2 * 256;
   			stDataEjector1To16[13].iSystemVacuum:= iBuffer1 OR iBuffer0;
   			iBuffer0 := 0;
   			iBuffer1 := 0;
   			iStep := iStep + 1;
   		END_IF;
   
   (* EPC-Value 1 *)
   	99:
   		siPDOData0.6 := 1;
   		siPDOData0.7 := 0;
   		IF siPDIData0.5  THEN
   			stDataEjector1To16[13].siWarningByte := siPDIData1;
   			iBuffer0 := siPDIData3;
   			iBuffer1 := siPDIData2 * 256;
   			stDataEjector1To16[13].iEvacuationTimeT1 := iBuffer1 OR iBuffer0;
   			iBuffer0 := 0;
   			iBuffer1 := 0;
   			iStep := iStep + 1;
   		END_IF;
   
   (* intermediate step *)
   	100:
   		siPDOData0.6 := 0;
   		siPDOData0.7 := 0;
   		IF NOT siPDIData0.5  THEN
   			iStep := iStep + 1;
   		END_IF;
   
   (* EPC-Value 2 *)
   	101:
   		siPDOData0.6 := 0;
   		siPDOData0.7 := 1;
   		IF siPDIData0.5  THEN
   			iBuffer0 := siPDIData3;
   			iBuffer1 := siPDIData2 * 256;
   			stDataEjector1To16[13].iLastFreeFlowVacuum := iBuffer1 OR iBuffer0;
   			iBuffer0 := 0;
   			iBuffer1 := 0;
   			iStep := iStep + 1;
   		END_IF;
   
   (* intermediate step *)
   	102:
   		siPDOData0.6 := 0;
   		siPDOData0.7 := 0;
   		IF NOT siPDIData0.5  THEN
   			iStep := iStep + 1;
   		END_IF;
   
   (* EPC-Value 3 *)
   	103:
   		siPDOData0.6 := 1;
   		siPDOData0.7 := 1;
   		IF siPDIData0.5  THEN
   			stDataEjector1To16[13].siLeakageOfLastCycle := siPDIData1;
   			iBuffer0 := siPDIData3;
   			iBuffer1 := siPDIData2 * 256;
   			stDataEjector1To16[13].iAirConsumptionOfLastCyc := iBuffer1 OR iBuffer0;
   			iBuffer0 := 0;
   			iBuffer1 := 0;
   			iStep := iStep + 1;
   		END_IF;
   
   	104:
   		IF iNumberOfEjectors >= 15 THEN
   			iStep := iStep + 1;
   		ELSE
   			iStep:= 0;
   		END_IF;
   
   (* Ejector 15 *)
   	105:
   		siPDOData0.0:=1;
   		siPDOData0.1:=1;
   		siPDOData0.2:=1;
   		siPDOData0.3:=1;
   		siPDOData0.4:=0;
   
   (* EPC-Value 0 *)
   		siPDOData0.6 := 0;
   		siPDOData0.7 := 0;
   
   		IF NOT siPDIData0.5  THEN
   			stDataEjector1To16[14].siErrorByte := siPDIData1;
   			iBuffer0 := siPDIData3;
   			iBuffer1 := siPDIData2 * 256;
   			stDataEjector1To16[14].iSystemVacuum:= iBuffer1 OR iBuffer0;
   			iBuffer0 := 0;
   			iBuffer1 := 0;
   			iStep := iStep + 1;
   		END_IF;
   
   (* EPC-Value 1 *)
   	106:
   		siPDOData0.6 := 1;
   		siPDOData0.7 := 0;
   		IF siPDIData0.5  THEN
   			stDataEjector1To16[14].siWarningByte := siPDIData1;
   			iBuffer0 := siPDIData3;
   			iBuffer1 := siPDIData2 * 256;
   			stDataEjector1To16[14].iEvacuationTimeT1 := iBuffer1 OR iBuffer0;
   			iBuffer0 := 0;
   			iBuffer1 := 0;
   			iStep := iStep + 1;
   		END_IF;
   
   (* intermediate step *)
   	107:
   		siPDOData0.6 := 0;
   		siPDOData0.7 := 0;
   		IF NOT siPDIData0.5  THEN
   			iStep := iStep + 1;
   		END_IF;
   
   (* EPC-Value 2 *)
   	108:
   		siPDOData0.6 := 0;
   		siPDOData0.7 := 1;
   		IF siPDIData0.5  THEN
   			iBuffer0 := siPDIData3;
   			iBuffer1 := siPDIData2 * 256;
   			stDataEjector1To16[14].iLastFreeFlowVacuum := iBuffer1 OR iBuffer0;
   			iBuffer0 := 0;
   			iBuffer1 := 0;
   			iStep := iStep + 1;
   		END_IF;
   
   (* intermediate step *)
   	109:
   		siPDOData0.6 := 0;
   		siPDOData0.7 := 0;
   		IF NOT siPDIData0.5  THEN
   			iStep := iStep + 1;
   		END_IF;
   
   (* EPC-Value 3 *)
   	110:
   		siPDOData0.6 := 1;
   		siPDOData0.7 := 1;
   
   		IF siPDIData0.5  THEN
   			stDataEjector1To16[14].siLeakageOfLastCycle := siPDIData1;
   			iBuffer0 := siPDIData3;
   			iBuffer1 := siPDIData2 * 256;
   			stDataEjector1To16[14].iAirConsumptionOfLastCyc := iBuffer1 OR iBuffer0;
   			iBuffer0 := 0;
   			iBuffer1 := 0;
   			iStep := iStep + 1;
   		END_IF;
   
   	111:
   		IF iNumberOfEjectors = 16 THEN
   			iStep := iStep + 1;
   		ELSE
   			iStep:= 0;
   		END_IF;
   
   (* Ejector 16 *)
   	112:
   		siPDOData0.0:=0;
   		siPDOData0.1:=0;
   		siPDOData0.2:=0;
   		siPDOData0.3:=0;
   		siPDOData0.4:=1;
   
   (* EPC-Value 0 *)
   		siPDOData0.6 := 0;
   		siPDOData0.7 := 0;
   		IF NOT siPDIData0.5  THEN
   			stDataEjector1To16[15].siErrorByte := siPDIData1;
   			iBuffer0 := siPDIData3;
   			iBuffer1 := siPDIData2 * 256;
   			stDataEjector1To16[15].iSystemVacuum:= iBuffer1 OR iBuffer0;
   			iBuffer0 := 0;
   			iBuffer1 := 0;
   			iStep := iStep + 1;
   		END_IF;
   
   (* EPC-Value 1 *)
   	113:
   		siPDOData0.6 := 1;
   		siPDOData0.7 := 0;
   		IF siPDIData0.5  THEN
   			stDataEjector1To16[15].siWarningByte := siPDIData1;
   			iBuffer0 := siPDIData3;
   			iBuffer1 := siPDIData2 * 256;
   			stDataEjector1To16[15].iEvacuationTimeT1 := iBuffer1 OR iBuffer0;
   			iBuffer0 := 0;
   			iBuffer1 := 0;
   			iStep := iStep + 1;
   		END_IF;
   
   (* intermediate step *)
   	114:
   		siPDOData0.6 := 0;
   		siPDOData0.7 := 0;
   		IF NOT siPDIData0.5  THEN
   			iStep := iStep + 1;
   		END_IF;
   
   (* EPC-Value 2 *)
   	115:
   		siPDOData0.6 := 0;
   		siPDOData0.7 := 1;
   		IF siPDIData0.5  THEN
   			iBuffer0 := siPDIData3;
   			iBuffer1 := siPDIData2 * 256;
   			stDataEjector1To16[15].iLastFreeFlowVacuum := iBuffer1 OR iBuffer0;
   			iBuffer0 := 0;
   			iBuffer1 := 0;
   			iStep := iStep + 1;
   		END_IF;
   
   (* intermediate step *)
   	116:
   		siPDOData0.6 := 0;
   		siPDOData0.7 := 0;
   		IF NOT siPDIData0.5  THEN
   			iStep := iStep + 1;
   		END_IF;
   
   (* EPC-Value 3 *)
   	117:
   		siPDOData0.6 := 1;
   		siPDOData0.7 := 1;
   		IF siPDIData0.5  THEN
   			stDataEjector1To16[15].siLeakageOfLastCycle := siPDIData1;
   			iBuffer0 := siPDIData3;
   			iBuffer1 := siPDIData2 * 256;
   			stDataEjector1To16[15].iAirConsumptionOfLastCyc := iBuffer1 OR iBuffer0;
   			iBuffer0 := 0;
   			iBuffer1 := 0;
   			iStep := iStep + 1;
   		END_IF;
   
   	118:
   		iStep := iStep + 1;
   
   (* Go to CU*)
   	119:
   		iStep:= 0;
   
   	END_CASE;
   
   (*Read feedback from ejectors 1-4*)
   	stDataEjector1To16[0].bAirSavingFunktion_H1 := siPDIData4.0;
   	stDataEjector1To16[0].bPartPresent_H2 := siPDIData4.1;
   	stDataEjector1To16[1].bAirSavingFunktion_H1 := siPDIData4.2;
   	stDataEjector1To16[1].bPartPresent_H2 := siPDIData4.3;
   	stDataEjector1To16[2].bAirSavingFunktion_H1 := siPDIData4.4;
   	stDataEjector1To16[2].bPartPresent_H2 := siPDIData4.5;
   	stDataEjector1To16[3].bAirSavingFunktion_H1 := siPDIData4.6;
   	stDataEjector1To16[3].bPartPresent_H2 := siPDIData4.7;
   
   (*Read feedback from ejectors 5-8*)
   	stDataEjector1To16[4].bAirSavingFunktion_H1 := siPDIData5.0;
   	stDataEjector1To16[4].bPartPresent_H2 := siPDIData5.1;
   	stDataEjector1To16[5].bAirSavingFunktion_H1 := siPDIData5.2;
   	stDataEjector1To16[5].bPartPresent_H2 := siPDIData5.3;
   	stDataEjector1To16[6].bAirSavingFunktion_H1 := siPDIData5.4;
   	stDataEjector1To16[6].bPartPresent_H2 := siPDIData5.5;
   	stDataEjector1To16[7].bAirSavingFunktion_H1 := siPDIData5.6;
   	stDataEjector1To16[7].bPartPresent_H2 := siPDIData5.7;
   
   (*Read feedback from ejectors 9-12*)
   	stDataEjector1To16[8].bAirSavingFunktion_H1 := siPDIData6.0;
   	stDataEjector1To16[8].bPartPresent_H2 := siPDIData6.1;
   	stDataEjector1To16[9].bAirSavingFunktion_H1 := siPDIData6.2;
   	stDataEjector1To16[9].bPartPresent_H2 := siPDIData6.3;
   	stDataEjector1To16[10].bAirSavingFunktion_H1 := siPDIData6.4;
   	stDataEjector1To16[10].bPartPresent_H2 := siPDIData6.5;
   	stDataEjector1To16[11].bAirSavingFunktion_H1 := siPDIData6.6;
   	stDataEjector1To16[11].bPartPresent_H2 := siPDIData6.7;
   
   (*Read feedback from ejectors 13-16*)
   	stDataEjector1To16[12].bAirSavingFunktion_H1 := siPDIData7.0;
   	stDataEjector1To16[12].bPartPresent_H2 := siPDIData7.1;
   	stDataEjector1To16[13].bAirSavingFunktion_H1 := siPDIData7.2;
   	stDataEjector1To16[13].bPartPresent_H2 := siPDIData7.3;
   	stDataEjector1To16[14].bAirSavingFunktion_H1 := siPDIData7.4;
   	stDataEjector1To16[14].bPartPresent_H2 := siPDIData7.5;
   	stDataEjector1To16[15].bAirSavingFunktion_H1 := siPDIData7.6;
   	stDataEjector1To16[15].bPartPresent_H2 := siPDIData7.7;
   
   (*Write Inputpressure from ext sensor*)
   	siPDOData1 := iInputPressure/100;
   
   (*Write Device Status Green*)
   	IF NOT siPDIData0.6 AND NOT   siPDIData0.7 THEN
   		bDeviceStateGreen :=   1;
   	ELSE
   		bDeviceStateGreen :=   0;
   	END_IF;
   
   (*Write Device Status Yellow*)
   	IF  siPDIData0.6 AND NOT   siPDIData0.7 THEN
   		bDeviceStateYellow :=   1;
   	ELSE
   		bDeviceStateYellow :=   0;
   	END_IF;
   
   (*Write Device Status Orange*)
   	IF  NOT siPDIData0.6 AND  siPDIData0.7 THEN
   		bDeviceStateOrange :=   1;
   	ELSE
   		bDeviceStateOrange :=   0;
   	END_IF;
   
   (*Write Device Status Red*)
   	IF   siPDIData0.6 AND  siPDIData0.7 THEN
   		bDeviceStateRed :=   1;
   	ELSE
   		bDeviceStateRed :=   0;
   	END_IF;
   
   (*Write control-bits for ejector 1 *)
   	IF iValveTypes.0 THEN (*NO*)
   		siPDOData2.0 :=  NOT bVacOnEjector1;
   		siPDOData2.1 := bBlowOffEjector1;
   	ELSE (*NC*)
   		siPDOData2.0 :=  bVacOnEjector1;
   		siPDOData2.1 := bBlowOffEjector1;
   	END_IF;
   
   (*Write control-bits for ejector 2 *)
   	IF iValveTypes.1 THEN (*NO*)
   		siPDOData2.2 :=  NOT bVacOnEjector2;
   		siPDOData2.3 := bBlowOffEjector2;
   	ELSE (*NC*)
   		siPDOData2.2 :=  bVacOnEjector2;
   		siPDOData2.3 := bBlowOffEjector2;
   	END_IF;
   
   (*Write control-bits for ejector 3 *)
   	IF iValveTypes.2 THEN (*NO*)
   		siPDOData2.4 :=  NOT bVacOnEjector3;
   		siPDOData2.5 := bBlowOffEjector3;
   	ELSE (*NC*)
   		siPDOData2.4 :=  bVacOnEjector3;
   		siPDOData2.5 := bBlowOffEjector3;
   	END_IF;
   
   (*Write control-bits for ejector 4 *)
   	IF iValveTypes.3 THEN (*NO*)
   		siPDOData2.6 :=  NOT bVacOnEjector4;
   		siPDOData2.7 := bBlowOffEjector4;
   	ELSE (*NC*)
   		siPDOData2.6 :=  bVacOnEjector4;
   		siPDOData2.7 := bBlowOffEjector4;
   	END_IF;
   
   (*Write control-bits for ejector 5 *)
   	IF iValveTypes.4 THEN (*NO*)
   		siPDOData3.0 :=  NOT bVacOnEjector5;
   		siPDOData3.1 := bBlowOffEjector5;
   	ELSE (*NC*)
   		siPDOData3.0 :=  bVacOnEjector5;
   		siPDOData3.1 := bBlowOffEjector5;
   	END_IF;
   
   (*Write control-bits for ejector 6 *)
   	IF iValveTypes.5 THEN (*NO*)
   		siPDOData3.2 :=  NOT bVacOnEjector6;
   		siPDOData3.3 := bBlowOffEjector6;
   	ELSE (*NC*)
   		siPDOData3.2 :=  bVacOnEjector6;
   		siPDOData3.3 := bBlowOffEjector6;
   	END_IF;
   
   (*Write control-bits for ejector 7 *)
   	IF iValveTypes.6 THEN (*NO*)
   		siPDOData3.4 :=  NOT bVacOnEjector7;
   		siPDOData3.5 := bBlowOffEjector7;
   	ELSE (*NC*)
   		siPDOData3.4 :=  bVacOnEjector7;
   		siPDOData3.5 := bBlowOffEjector7;
   	END_IF;
   
   (*Write control-bits for ejector 8 *)
   	IF iValveTypes.7 THEN (*NO*)
   		siPDOData3.6 :=  NOT bVacOnEjector8;
   		siPDOData3.7 := bBlowOffEjector8;
   	ELSE (*NC*)
   		siPDOData3.6 :=  bVacOnEjector8;
   		siPDOData3.7 := bBlowOffEjector8;
   	END_IF;
   
   (*Write control-bits for ejector 9 *)
   	IF iValveTypes.8 THEN (*NO*)
   		siPDOData4.0 :=  NOT bVacOnEjector9;
   		siPDOData4.1 := bBlowOffEjector9;
   	ELSE (*NC*)
   		siPDOData4.0 :=  bVacOnEjector9;
   		siPDOData4.1 := bBlowOffEjector9;
   	END_IF;
   
   (*Write control-bits for ejector 10 *)
   	IF iValveTypes.9 THEN (*NO*)
   		siPDOData4.2 :=  NOT bVacOnEjector10;
   		siPDOData4.3 := bBlowOffEjector10;
   	ELSE (*NC*)
   		siPDOData4.2 :=  bVacOnEjector10;
   		siPDOData4.3 := bBlowOffEjector10;
   	END_IF;
   
   (*Write control-bits for ejector 11*)
   	IF iValveTypes.10 THEN (*NO*)
   		siPDOData4.4 :=  NOT bVacOnEjector11;
   		siPDOData4.5 := bBlowOffEjector11;
   	ELSE (*NC*)
   		siPDOData4.4 :=  bVacOnEjector11;
   		siPDOData4.5 := bBlowOffEjector11;
   	END_IF;
   
   (*Write control-bits for ejector 12 *)
   	IF iValveTypes.11 THEN (*NO*)
   		siPDOData4.6 :=  NOT bVacOnEjector12;
   		siPDOData4.7 := bBlowOffEjector12;
   	ELSE (*NC*)
   		siPDOData4.6 :=  bVacOnEjector12;
   		siPDOData4.7 := bBlowOffEjector12;
   	END_IF;
   
   (*Write control-bits for ejector 13 *)
   	IF iValveTypes.12 THEN (*NO*)
   		siPDOData5.0 :=  NOT bVacOnEjector13;
   		siPDOData5.1 := bBlowOffEjector13;
   	ELSE (*NC*)
   		siPDOData5.0 :=  bVacOnEjector13;
   		siPDOData5.1 := bBlowOffEjector13;
   	END_IF;
   
   (*Write control-bits for ejector 14 *)
   	IF iValveTypes.13 THEN (*NO*)
   		siPDOData5.2 :=  NOT bVacOnEjector14;
   		siPDOData5.3 := bBlowOffEjector14;
   	ELSE (*NC*)
   		siPDOData5.2 :=  bVacOnEjector14;
   		siPDOData5.3 := bBlowOffEjector14;
   	END_IF;
   
   (*Write control-bits for ejector 15 *)
   	IF iValveTypes.14 THEN (*NO*)
   		siPDOData5.4 :=  NOT bVacOnEjector15;
   		siPDOData5.5 := bBlowOffEjector15;
   	ELSE (*NC*)
   		siPDOData5.4 :=  bVacOnEjector15;
   		siPDOData5.5 := bBlowOffEjector15;
   	END_IF;
   
   (*Write control-bits for ejector 16 *)
   	IF iValveTypes.15 THEN (*NO*)
   		siPDOData5.6 :=  NOT bVacOnEjector16;
   		siPDOData5.7 := bBlowOffEjector16;
   	ELSE (*NC*)
   		siPDOData5.6 :=  bVacOnEjector16;
   		siPDOData5.7 := bBlowOffEjector16;
   	END_IF;
   END_IF;
   EnableOut := EnableIn;
   
END_ROUTINE
END_ADD_ON_INSTRUCTION
